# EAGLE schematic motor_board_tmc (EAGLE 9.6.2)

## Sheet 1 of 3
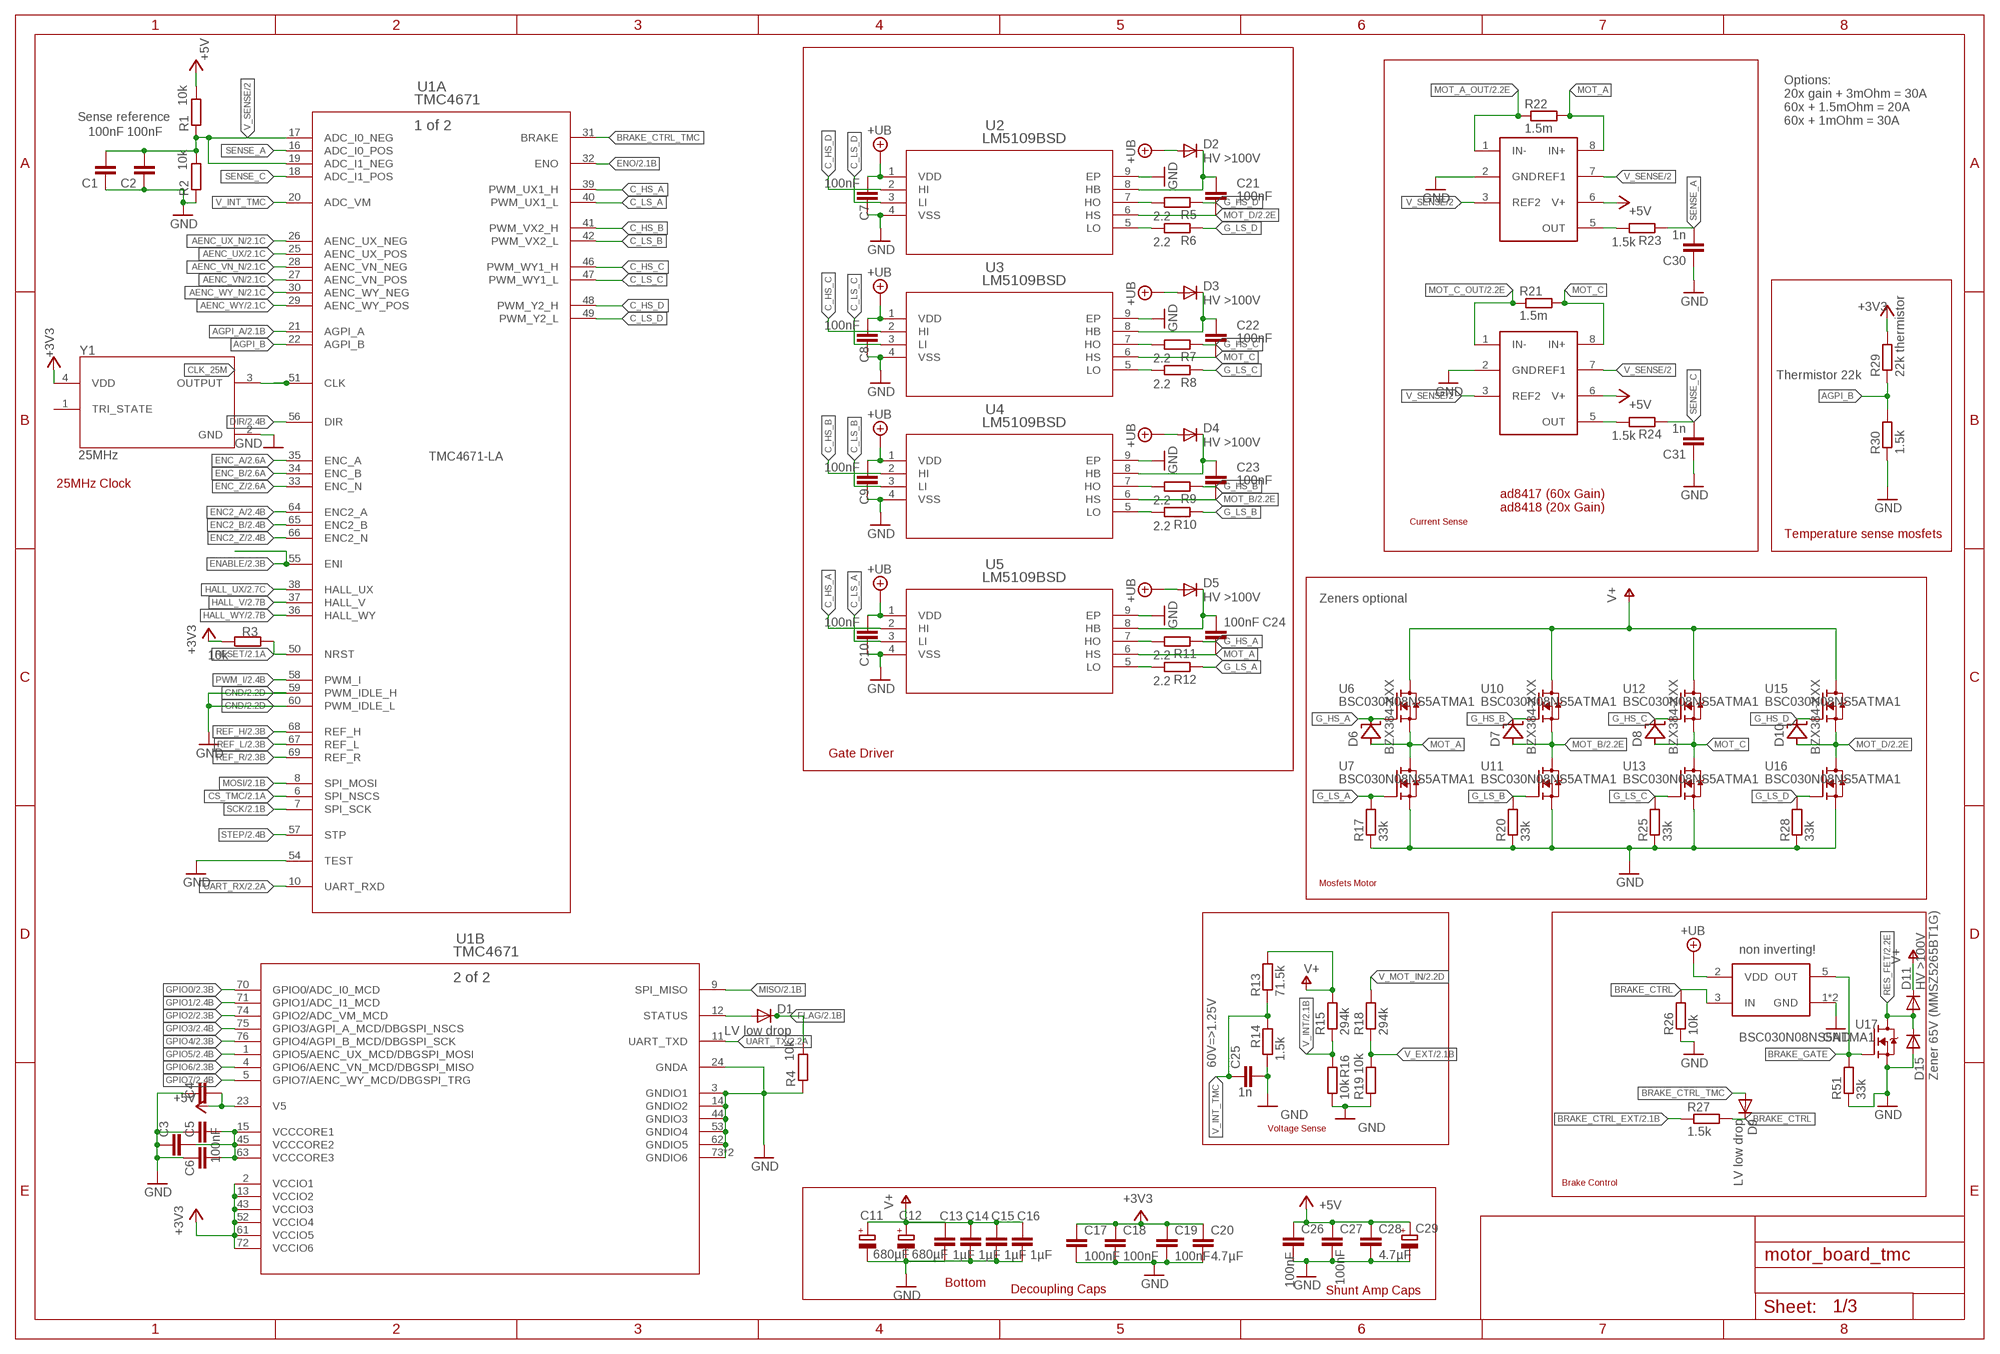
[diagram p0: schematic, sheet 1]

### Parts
C1  100nF  C-EUC0603  [C0603]
C2  100nF  C-EUC0603  [C0603]
C3  100nF  C-EUC0603  [C0603]
C4  100nF  C-EUC0603  [C0603]
C5  100nF  C-EUC0603  [C0603]
C6  100nF  C-EUC0603  [C0603]
C7  100nF  C-EUC0603  [C0603]
C8  100nF  C-EUC0603  [C0603]
C9  100nF  C-EUC0603  [C0603]
C10  100nF  C-EUC0603  [C0603]
C11  680µF  CPOL-EUE7.5-16  [E7,5-16]
C12  680µF  CPOL-EUE7.5-16  [E7,5-16]
C13  1µF  C-EUC1206  [C1206]
C14  1µF  C-EUC1206  [C1206]
C15  1µF  C-EUC1206  [C1206]
C16  1µF  C-EUC1206  [C1206]
C17  100nF  C-EUC0603  [C0603]
C18  100nF  C-EUC0603  [C0603]
C19  100nF  C-EUC0603  [C0603]
C20  4.7µF  C-EUC0805  [C0805]
C21  100nF  C-EUC0805  [C0805]
C22  100nF  C-EUC0805  [C0805]
C23  100nF  C-EUC0805  [C0805]
C24  100nF  C-EUC0805  [C0805]
C25  1n  C-EUC0603  [C0603]
C26  100nF  C-EUC0603  [C0603]
C27  100nF  C-EUC0603  [C0603]
C28  4.7µF  C-EUC0805  [C0805]
C29  CPOL-EUE5-8.5  [E5-8,5]
C30  1n  C-EUC0603  [C0603]
C31  1n  C-EUC0603  [C0603]
D1  LV low drop  DIODE_SOD-123FL  [SOD-123FL]
D2  HV >100V  DIODE_SOD-123FL  [SOD-123FL]
D3  HV >100V  DIODE_SOD-123FL  [SOD-123FL]
D4  HV >100V  DIODE_SOD-123FL  [SOD-123FL]
D5  HV >100V  DIODE_SOD-123FL  [SOD-123FL]
D6  BZX384-XXX  [SOD323-R]
D7  BZX384-XXX  [SOD323-R]
D8  BZX384-XXX  [SOD323-R]
D9  LV low drop  DIODE_SOD-123FL  [SOD-123FL]
D10  BZX384-XXX  [SOD323-R]
D11  HV >100V  DIODE_SOD-123FL  [SOD-123FL]
D15  Zener 65V (MMSZ5265BT1G)  DIODE_SOD-123FL  [SOD-123FL]
R1  10k  R-EU_R0603  [R0603]
R2  10k  R-EU_R0603  [R0603]
R3  10k  R-EU_R0603  [R0603]
R4  10k  R-EU_R0603  [R0603]
R5  2.2  R-EU_R0603  [R0603]
R6  2.2  R-EU_R0603  [R0603]
R7  2.2  R-EU_R0603  [R0603]
R8  2.2  R-EU_R0603  [R0603]
R9  2.2  R-EU_R0603  [R0603]
R10  2.2  R-EU_R0603  [R0603]
R11  2.2  R-EU_R0603  [R0603]
R12  2.2  R-EU_R0603  [R0603]
R13  71.5k  R-EU_R0805  [R0805]
R14  1.5k  R-EU_R0603  [R0603]
R15  294k  R-EU_R0805  [R0805]
R16  10k  R-EU_R0603  [R0603]
R17  33k  R-EU_R0603  [R0603]
R18  294k  R-EU_R0805  [R0805]
R19  10k  R-EU_R0603  [R0603]
R20  33k  R-EU_R0603  [R0603]
R21  1.5m  R-EU_R2512  [R2512]
R22  1.5m  R-EU_R2512  [R2512]
R23  1.5k  R-EU_R0603  [R0603]
R24  1.5k  R-EU_R0603  [R0603]
R25  33k  R-EU_R0603  [R0603]
R26  10k  R-EU_R0603  [R0603]
R27  1.5k  R-EU_R0603  [R0603]
R28  33k  R-EU_R0603  [R0603]
R29  22k thermistor  R-EU_R0603  [R0603]
R30  1.5k  R-EU_R0603  [R0603]
R51  33k  R-EU_R0603  [R0603]
U1  TMC4671  [QFN76_10P5X6P5]
U2  LM5109BSD  [SDC08A]
U3  LM5109BSD  [SDC08A]
U4  LM5109BSD  [SDC08A]
U5  LM5109BSD  [SDC08A]
U6  BSC030N08NS5ATMA1  [MOSFET_BSC093N04LSGATMA1]
U7  BSC030N08NS5ATMA1  [MOSFET_BSC093N04LSGATMA1]
U8  AD841X  [MSOP8]
U9  AD841X  [MSOP8]
U10  BSC030N08NS5ATMA1  [MOSFET_BSC093N04LSGATMA1]
U11  BSC030N08NS5ATMA1  [MOSFET_BSC093N04LSGATMA1]
U12  BSC030N08NS5ATMA1  [MOSFET_BSC093N04LSGATMA1]
U13  BSC030N08NS5ATMA1  [MOSFET_BSC093N04LSGATMA1]
U14  MCP14XX  [SOT23-5L]
U15  BSC030N08NS5ATMA1  [MOSFET_BSC093N04LSGATMA1]
U16  BSC030N08NS5ATMA1  [MOSFET_BSC093N04LSGATMA1]
U17  BSC030N08NS5ATMA1  [MOSFET_BSC093N04LSGATMA1]
Y1  25MHz  ECS-327KE-TR  [ECS-327KE-TR]

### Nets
+3V3: C17.1 C18.1 C19.1 C20.1 R3.2 R29.2 U1.2(B:VCCIO1) U1.13(B:VCCIO2) U1.43(B:VCCIO3) U1.52(B:VCCIO4) U1.61(B:VCCIO5) U1.72(B:VCCIO6) Y1.4(VDD) ; also sheet 2,3
+5V: C4.2 C26.1 C27.1 C28.1 C29.+ R1.2 U1.23(B:V5) U8.6(V+) U9.6(V+) ; also sheet 2,3
AENC_UX: U1.25(A:AENC_UX_POS) ; also sheet 2
AENC_UX_N: U1.26(A:AENC_UX_NEG) ; also sheet 2
AENC_VN: U1.27(A:AENC_VN_POS) ; also sheet 2
AENC_VN_N: U1.28(A:AENC_VN_NEG) ; also sheet 2
AENC_WY: U1.29(A:AENC_WY_POS) ; also sheet 2
AENC_WY_N: U1.30(A:AENC_WY_NEG) ; also sheet 2
AGPI_A: U1.21(A:AGPI_A) ; also sheet 2
AGPI_B: R29.1 R30.2 U1.22(A:AGPI_B)
BRAKE_CTRL: D9.C R26.2 R27.2 U14.3(IN)
BRAKE_CTRL_EXT: R27.1 ; also sheet 2
BRAKE_CTRL_TMC: D9.A U1.31(A:BRAKE)
BRAKE_GATE: R51.2 U14.5(OUT) U17.4(G)
C_HS_A: U1.39(A:PWM_UX1_H) U5.2(HI)
C_HS_B: U1.41(A:PWM_VX2_H) U4.2(HI)
C_HS_C: U1.46(A:PWM_WY1_H) U3.2(HI)
C_HS_D: U1.48(A:PWM_Y2_H) U2.2(HI)
C_LS_A: U1.40(A:PWM_UX1_L) U5.3(LI)
C_LS_B: U1.42(A:PWM_VX2_L) U4.3(LI)
C_LS_C: U1.47(A:PWM_WY1_L) U3.3(LI)
C_LS_D: U1.49(A:PWM_Y2_L) U2.3(LI)
CLK_25M: U1.51(A:CLK) Y1.3(OUTPUT)
CS_TMC: U1.6(A:SPI_NSCS) ; also sheet 2
DIR: U1.56(A:DIR) ; also sheet 2
ENABLE: U1.55(A:ENI) ; also sheet 2
ENC2_A: U1.64(A:ENC2_A) ; also sheet 2
ENC2_B: U1.65(A:ENC2_B) ; also sheet 2
ENC2_Z: U1.66(A:ENC2_N) ; also sheet 2
ENC_A: U1.35(A:ENC_A) ; also sheet 2
ENC_B: U1.34(A:ENC_B) ; also sheet 2
ENC_Z: U1.33(A:ENC_N) ; also sheet 2
ENO: U1.32(A:ENO) ; also sheet 2
FLAG: D1.C R4.2 ; also sheet 2
G_HS_A: D6.C R11.1 U6.4(G)
G_HS_B: D7.C R9.1 U10.4(G)
G_HS_C: D8.C R7.1 U12.4(G)
G_HS_D: D10.C R5.1 U15.4(G)
G_LS_A: R12.1 R17.2 U7.4(G)
G_LS_B: R10.1 R20.2 U11.4(G)
G_LS_C: R8.1 R25.2 U13.4(G)
G_LS_D: R6.1 R28.2 U16.4(G)
GND: C1.1 C2.1 C3.1 C4.1 C5.1 C6.1 C7.1 C8.1 C9.1 C10.1 C11.- C12.- C13.2 C14.2 C15.2 C16.2 C17.2 C18.2 C19.2 C20.2 C25.2 C26.2 C27.2 C28.2 C29.- C30.1 C31.1 D15.A R2.1 R4.1 R14.1 R16.1 R17.1 R19.1 R20.1 R25.1 R26.1 R28.1 R30.1 R51.1 U1.3(B:GNDIO1) U1.14(B:GNDIO2) U1.24(B:GNDA) U1.44(B:GNDIO3) U1.53(B:GNDIO4) U1.54(A:TEST) U1.59(A:PWM_IDLE_H) U1.60(A:PWM_IDLE_L) U1.62(B:GNDIO5) U1.73(B:GNDIO6) U1.77(B:GNDIO6) U2.4(VSS) U2.9(EP) U3.4(VSS) U3.9(EP) U4.4(VSS) U4.9(EP) U5.4(VSS) U5.9(EP) U7.1(S) U7.2(S) U7.3(S) U8.2(GND) U9.2(GND) U11.1(S) U11.2(S) U11.3(S) U13.1(S) U13.2(S) U13.3(S) U14.1(GND) U14.4(GND) U16.1(S) U16.2(S) U16.3(S) U17.1(S) U17.2(S) U17.3(S) Y1.2(GND) ; also sheet 2,3
GPIO0: U1.70(B:GPIO0/ADC_I0_MCD) ; also sheet 2
GPIO1: U1.71(B:GPIO1/ADC_I1_MCD) ; also sheet 2
GPIO2: U1.74(B:GPIO2/ADC_VM_MCD) ; also sheet 2
GPIO3: U1.75(B:GPIO3/AGPI_A_MCD/DBGSPI_NSCS) ; also sheet 2
GPIO4: U1.76(B:GPIO4/AGPI_B_MCD/DBGSPI_SCK) ; also sheet 2
GPIO5: U1.1(B:GPIO5/AENC_UX_MCD/DBGSPI_MOSI) ; also sheet 2
GPIO6: U1.4(B:GPIO6/AENC_VN_MCD/DBGSPI_MISO) ; also sheet 2
GPIO7: U1.5(B:GPIO7/AENC_WY_MCD/DBGSPI_TRG) ; also sheet 2
HALL_UX: U1.38(A:HALL_UX) ; also sheet 2
HALL_V: U1.37(A:HALL_V) ; also sheet 2
HALL_WY: U1.36(A:HALL_WY) ; also sheet 2
MISO: U1.9(B:SPI_MISO) ; also sheet 2
MOSI: U1.8(A:SPI_MOSI) ; also sheet 2
MOT_A: C24.2 D6.A R22.2 U5.6(HS) U6.1(S) U6.2(S) U6.3(S) U7.5(D) U8.8(IN+)
MOT_A_OUT: R22.1 U8.1(IN-) ; also sheet 2
MOT_B: C23.2 D7.A U4.6(HS) U10.1(S) U10.2(S) U10.3(S) U11.5(D) ; also sheet 2
MOT_C: C22.2 D8.A R21.2 U3.6(HS) U9.8(IN+) U12.1(S) U12.2(S) U12.3(S) U13.5(D)
MOT_C_OUT: R21.1 U9.1(IN-) ; also sheet 2
MOT_D: C21.2 D10.A U2.6(HS) U15.1(S) U15.2(S) U15.3(S) U16.5(D) ; also sheet 2
N$4: D1.A U1.12(B:STATUS)
N$6: R23.2 U8.5(OUT)
N$10: R24.2 U9.5(OUT)
N$13: R12.2 U5.5(LO)
N$18: C24.1 D5.C U5.8(HB)
N$27: R11.2 U5.7(HO)
N$28: C23.1 D4.C U4.8(HB)
N$29: R10.2 U4.5(LO)
N$30: R9.2 U4.7(HO)
N$31: C21.1 D2.C U2.8(HB)
N$32: R6.2 U2.5(LO)
N$33: R5.2 U2.7(HO)
N$34: C22.1 D3.C U3.8(HB)
N$35: R8.2 U3.5(LO)
N$36: R7.2 U3.7(HO)
PWM_I: U1.58(A:PWM_I) ; also sheet 2
REF_H: U1.68(A:REF_H) ; also sheet 2
REF_L: U1.67(A:REF_L) ; also sheet 2
REF_R: U1.69(A:REF_R) ; also sheet 2
RES_FET: D11.A D15.C U17.5(D) ; also sheet 2
RESET: R3.1 U1.50(A:NRST) ; also sheet 2
SCK: U1.7(A:SPI_SCK) ; also sheet 2
SENSE_A: C30.2 R23.1 U1.16(A:ADC_I0_POS)
SENSE_C: C31.2 R24.1 U1.18(A:ADC_I1_POS)
STEP: U1.57(A:STP) ; also sheet 2
UART_RX: U1.10(A:UART_RXD) ; also sheet 2
UART_TX: U1.11(B:UART_TXD) ; also sheet 2
V+: C11.+ C12.+ C13.1 C14.1 C15.1 C16.1 D11.C R13.2 R15.2 U6.5(D) U10.5(D) U12.5(D) U15.5(D) ; also sheet 2,3
V_EXT: R18.1 R19.2 ; also sheet 2
V_GD: C7.2 C8.2 C9.2 C10.2 D2.A D3.A D4.A D5.A U2.1(VDD) U3.1(VDD) U4.1(VDD) U5.1(VDD) U14.2(VDD) ; supply symbol labelled +UB ; also sheet 2,3
V_INT: R15.1 R16.2 ; also sheet 2
V_INT_TMC: C25.1 R13.1 R14.2 U1.20(A:ADC_VM)
V_MOT_IN: R18.2 ; also sheet 2,3
V_SENSE/2: C1.2 C2.2 R1.1 R2.2 U1.17(A:ADC_I0_NEG) U1.19(A:ADC_I1_NEG) U8.3(REF2) U8.7(REF1) U9.3(REF2) U9.7(REF1)
VCORE: C3.2 C5.2 C6.2 U1.15(B:VCCCORE1) U1.45(B:VCCCORE2) U1.63(B:VCCCORE3)
Unconnected: Y1.1(TRI_STATE)

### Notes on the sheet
- Sense reference
- Options:
  20x gain + 3mOhm = 30A
  60x + 1.5mOhm = 20A
  60x + 1mOhm = 30A
- Thermistor 22k
- TMC4671-LA
- 25MHz Clock
- Current Sense
- ad8417 (60x Gain)
  ad8418 (20x Gain)
- Temperature sense mosfets
- Zeners optional
- Gate Driver
- Mosfets Motor
- non inverting!
- 60V=>1.25V
- Voltage Sense
- Brake Control
- Bottom
- Decoupling Caps | Shunt Amp Caps

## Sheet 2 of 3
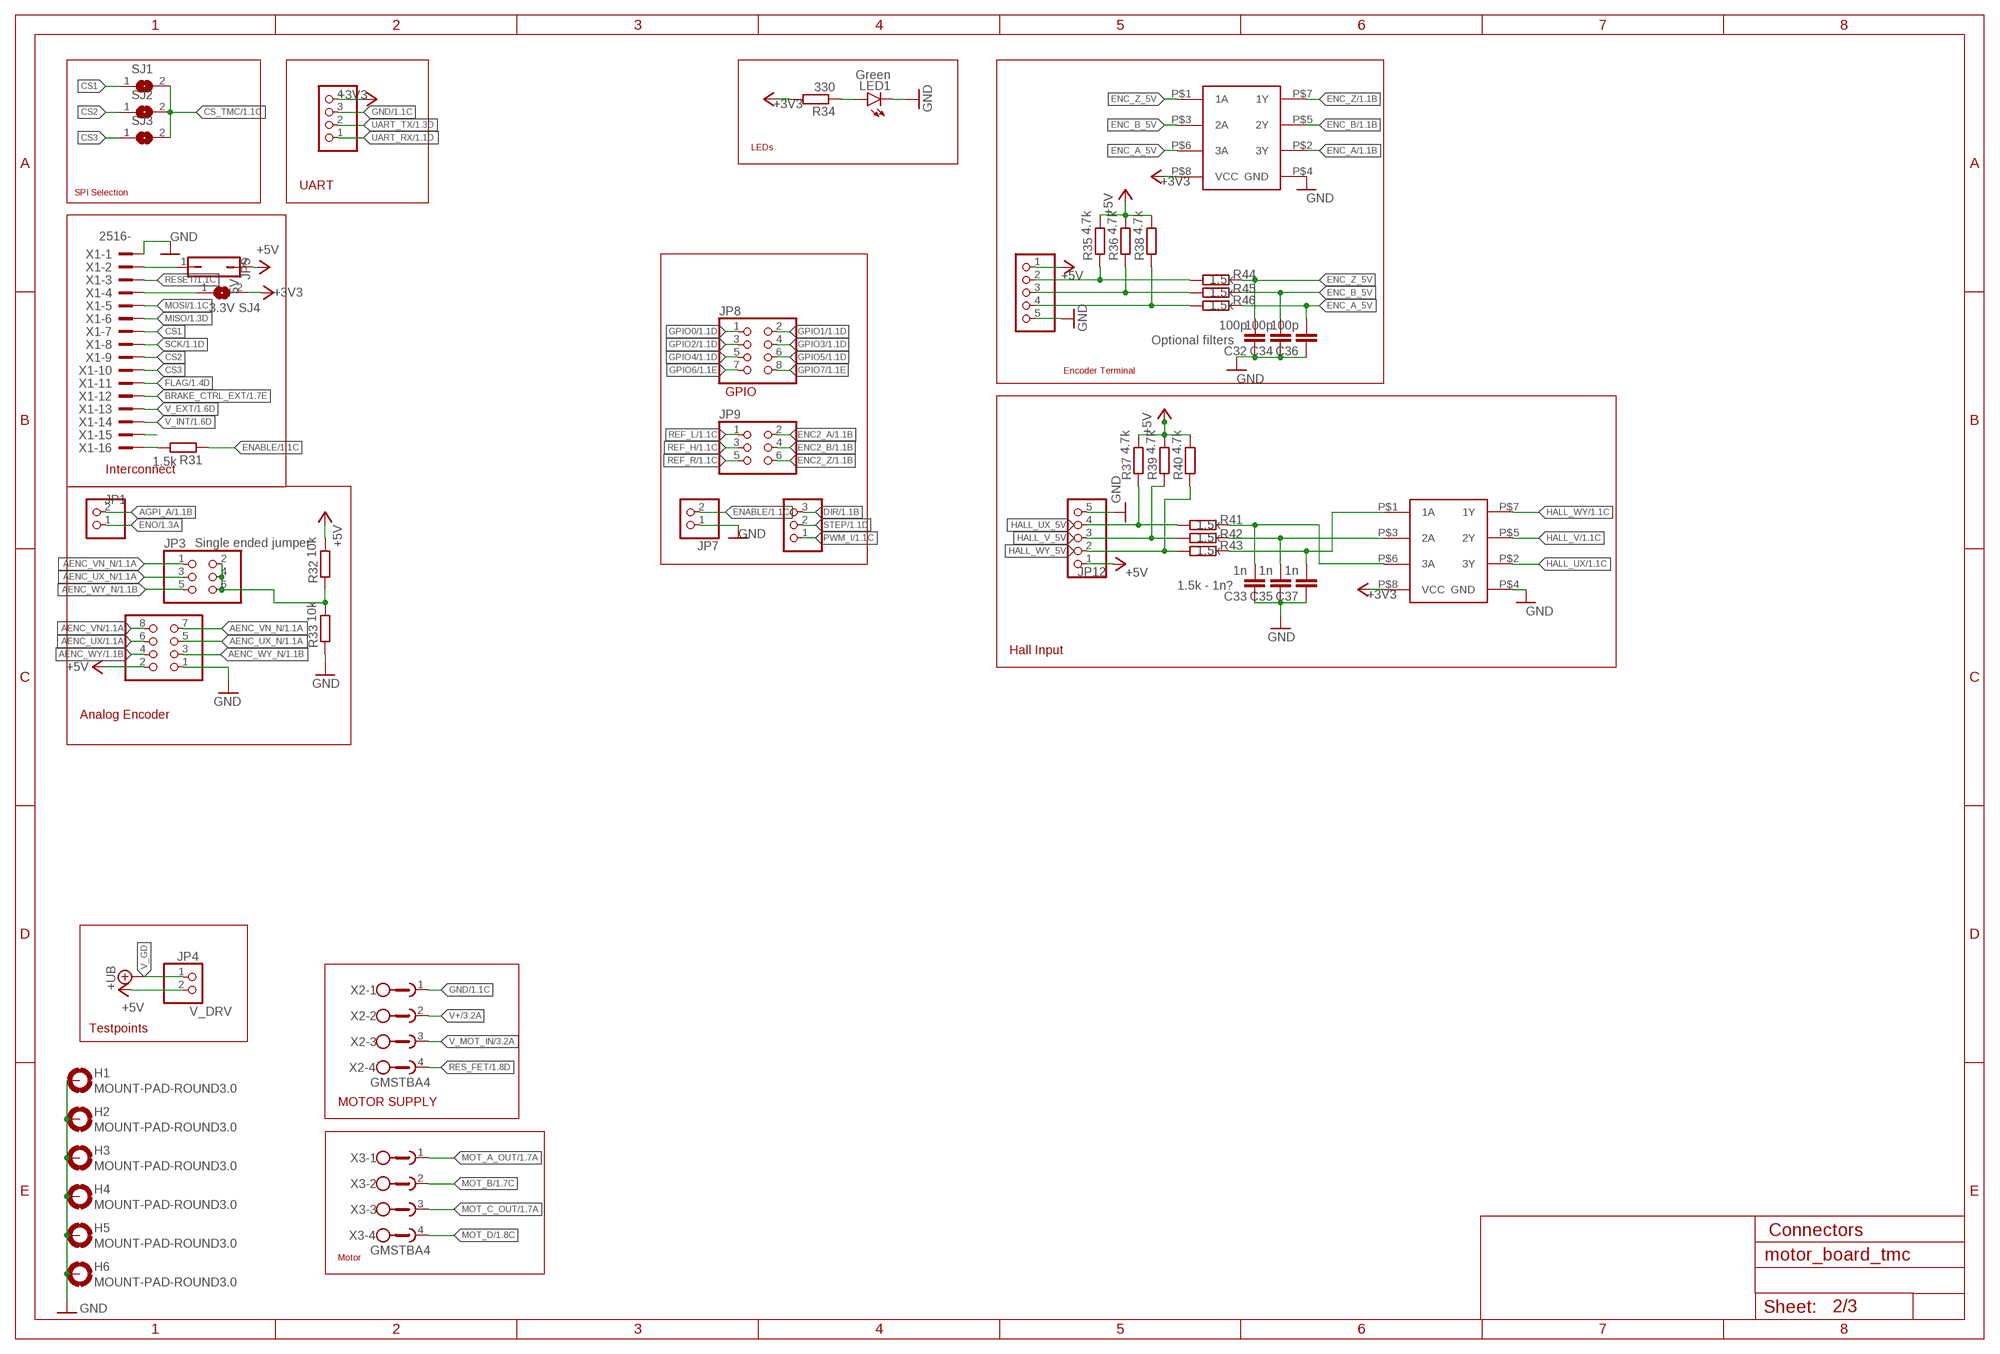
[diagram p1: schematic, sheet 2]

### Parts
C32  100p  C-EUC0603  [C0603]
C33  1n  C-EUC0603  [C0603]
C34  100p  C-EUC0603  [C0603]
C35  1n  C-EUC0603  [C0603]
C36  100p  C-EUC0603  [C0603]
C37  1n  C-EUC0603  [C0603]
H1  MOUNT-PAD-ROUND3.0  [3,0-PAD]
H2  MOUNT-PAD-ROUND3.0  [3,0-PAD]
H3  MOUNT-PAD-ROUND3.0  [3,0-PAD]
H4  MOUNT-PAD-ROUND3.0  [3,0-PAD]
H5  MOUNT-PAD-ROUND3.0  [3,0-PAD]
H6  MOUNT-PAD-ROUND3.0  [3,0-PAD]
JP1  PINHD-1X2  [1X02]
JP2  PINHD-2X4  [2X04]
JP3  PINHD-2X3  [2X03]
JP4  V_DRV  PINHD-1X2  [1X02]
JP5  5V  JP1Q  [JP1]
JP6  PINHD-1X4  [1X04]
JP7  PINHD-1X2  [1X02]
JP8  PINHD-2X4  [2X04]
JP9  PINHD-2X3  [2X03]
JP10  PINHD-1X3  [1X03]
JP11  PINHD-1X5  [1X05]
JP12  PINHD-1X5  [1X05]
LED1  Green  LEDSML0805  [SML0805]
R31  1.5k  R-EU_R0603  [R0603]
R32  10k  R-EU_R0603  [R0603]
R33  10k  R-EU_R0603  [R0603]
R34  330  R-EU_R0603  [R0603]
R35  4.7k  R-EU_R0603  [R0603]
R36  4.7k  R-EU_R0603  [R0603]
R37  4.7k  R-EU_R0603  [R0603]
R38  4.7k  R-EU_R0603  [R0603]
R39  4.7k  R-EU_R0603  [R0603]
R40  4.7k  R-EU_R0603  [R0603]
R41  1.5k  R-EU_R0603  [R0603]
R42  1.5k  R-EU_R0603  [R0603]
R43  1.5k  R-EU_R0603  [R0603]
R44  1.5k  R-EU_R0603  [R0603]
R45  1.5k  R-EU_R0603  [R0603]
R46  1.5k  R-EU_R0603  [R0603]
SJ1  SJ  [SJ]
SJ2  SJ  [SJ]
SJ3  SJ  [SJ]
SJ4  3.3V  SJ  [SJ]
U18  NC7NZ17K8X-3-BUFFER  [VFSOP-8]
U19  NC7NZ17K8X-3-BUFFER  [VFSOP-8]
X1  2516-  [PAK100/2500-16]
X2  GMSTBA4  [GMSTBA4]
X3  GMSTBA4  [GMSTBA4]

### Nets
+3V3: JP6.4 R34.2 SJ4.2 U18.P$8(VCC) U19.P$8(VCC) ; also sheet 1,3
+5V: JP2.2 JP4.2 JP5.2 JP11.1 JP12.1 R32.2 R35.2 R36.2 R37.2 R38.2 R39.2 R40.2 ; also sheet 1,3
AENC_UX: JP2.6 ; also sheet 1
AENC_UX_N: JP2.5 JP3.3 ; also sheet 1
AENC_VN: JP2.8 ; also sheet 1
AENC_VN_N: JP2.7 JP3.1 ; also sheet 1
AENC_WY: JP2.4 ; also sheet 1
AENC_WY_N: JP2.3 JP3.5 ; also sheet 1
AGPI_A: JP1.2 ; also sheet 1
BRAKE_CTRL_EXT: X1.12 ; also sheet 1
CS1: SJ1.1 X1.7
CS2: SJ2.1 X1.9
CS3: SJ3.1 X1.10
CS_TMC: SJ1.2 SJ2.2 SJ3.2 ; also sheet 1
DIR: JP10.3 ; also sheet 1
ENABLE: JP7.2 R31.1 ; also sheet 1
ENC2_A: JP9.2 ; also sheet 1
ENC2_B: JP9.4 ; also sheet 1
ENC2_Z: JP9.6 ; also sheet 1
ENC_A: U18.P$2(3Y) ; also sheet 1
ENC_A_5V: C36.2 R46.1 U18.P$6(3A)
ENC_B: U18.P$5(2Y) ; also sheet 1
ENC_B_5V: C34.2 R45.1 U18.P$3(2A)
ENC_Z: U18.P$7(1Y) ; also sheet 1
ENC_Z_5V: C32.2 R44.1 U18.P$1(1A)
ENO: JP1.1 ; also sheet 1
FLAG: X1.11 ; also sheet 1
GND: C32.1 C33.1 C34.1 C35.1 C36.1 C37.1 H1.B3,0(MOUNT) H2.B3,0(MOUNT) H3.B3,0(MOUNT) H4.B3,0(MOUNT) H5.B3,0(MOUNT) H6.B3,0(MOUNT) JP2.1 JP6.3 JP7.1 JP11.5 JP12.5 LED1.C R33.1 U18.P$4(GND) U19.P$4(GND) X1.1 X2.1 ; also sheet 1,3
GPIO0: JP8.1 ; also sheet 1
GPIO1: JP8.2 ; also sheet 1
GPIO2: JP8.3 ; also sheet 1
GPIO3: JP8.4 ; also sheet 1
GPIO4: JP8.5 ; also sheet 1
GPIO5: JP8.6 ; also sheet 1
GPIO6: JP8.7 ; also sheet 1
GPIO7: JP8.8 ; also sheet 1
HALL_UX: U19.P$2(3Y) ; also sheet 1
HALL_UX_5V: C33.2 R41.1 U19.P$6(3A)
HALL_V: U19.P$5(2Y) ; also sheet 1
HALL_V_5V: C35.2 R42.1 U19.P$3(2A)
HALL_WY: U19.P$7(1Y) ; also sheet 1
HALL_WY_5V: C37.2 R43.1 U19.P$1(1A)
MISO: X1.6 ; also sheet 1
MOSI: X1.5 ; also sheet 1
MOT_A_OUT: X3.1 ; also sheet 1
MOT_B: X3.2 ; also sheet 1
MOT_C_OUT: X3.3 ; also sheet 1
MOT_D: X3.4 ; also sheet 1
N$1: JP12.4 R37.1 R41.2
N$2: X1.15
N$3: JP12.3 R39.1 R42.2
N$7: JP11.4 R38.1 R46.2
N$8: LED1.A R34.1
N$9: JP11.3 R36.1 R45.2
N$11: JP11.2 R35.1 R44.2
N$15: JP12.2 R40.1 R43.2
N$17: R31.2 X1.16
N$20: SJ4.1 X1.4
N$22: JP3.2 JP3.4 JP3.6 R32.1 R33.2
N$23: JP5.1 X1.2
PWM_I: JP10.1 ; also sheet 1
REF_H: JP9.3 ; also sheet 1
REF_L: JP9.1 ; also sheet 1
REF_R: JP9.5 ; also sheet 1
RES_FET: X2.4 ; also sheet 1
RESET: X1.3 ; also sheet 1
SCK: X1.8 ; also sheet 1
STEP: JP10.2 ; also sheet 1
UART_RX: JP6.1 ; also sheet 1
UART_TX: JP6.2 ; also sheet 1
V+: X2.2 ; also sheet 1,3
V_EXT: X1.13 ; also sheet 1
V_GD: JP4.1 ; supply symbol labelled +UB ; also sheet 1,3
V_INT: X1.14 ; also sheet 1
V_MOT_IN: X2.3 ; also sheet 1,3

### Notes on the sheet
- LEDs
- UART
- SPI Selection
- Optional filters
- Encoder Terminal
- GPIO
- Interconnect
- Single ended jumper
- 1.5k - 1n?
- Hall Input
- Analog Encoder
- Testpoints
- MOTOR SUPPLY
- Connectors
- Motor

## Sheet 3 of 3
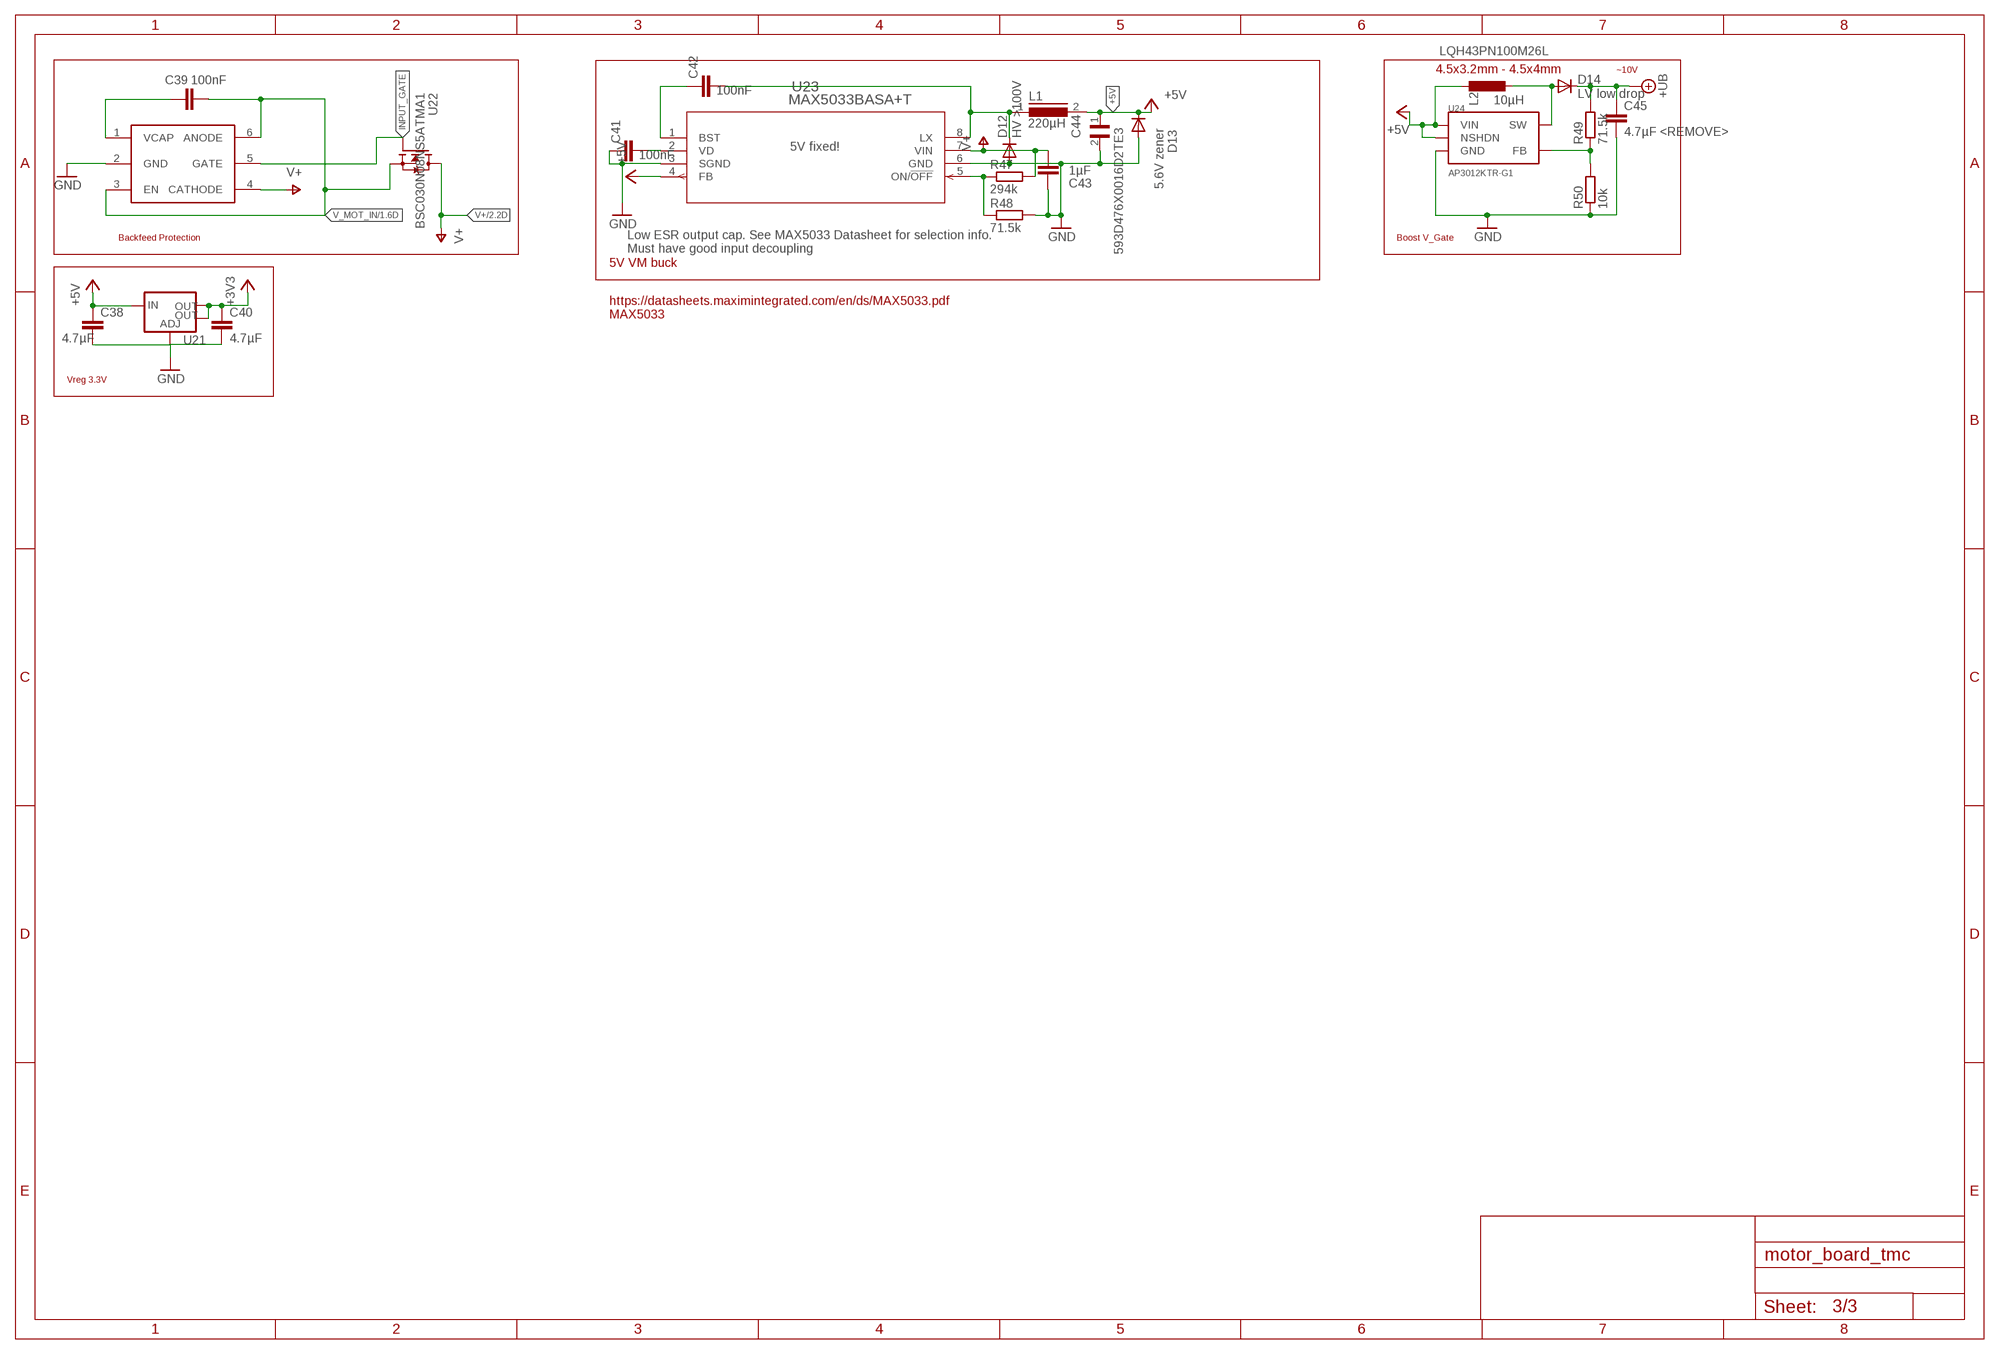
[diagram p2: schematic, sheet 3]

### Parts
C38  4.7µF  C-EUC0805  [C0805]
C39  100nF  C-EUC0805  [C0805]
C40  4.7µF  C-EUC0805  [C0805]
C41  100nF  C-EUC0603  [C0603]
C42  100nF  C-EUC0603  [C0603]
C43  1µF  C-EUC1206  [C1206]
C44  593D476X0016D2TE3  [CAPPM7343X310N]
C45  4.7µF <REMOVE>  C-EUC0805  [C0805]
D12  HV >100V  DIODE_SOD-123FL  [SOD-123FL]
D13  5.6V zener  DIODE_SOD-123FL  [SOD-123FL]
D14  LV low drop  DIODE_SOD-123FL  [SOD-123FL]
L1  220µH  8MMINDUCTOR  [8MMINDUCTOR]
L2  10µH  L-EUL4532P  [L4532P]
R47  294k  R-EU_R0805  [R0805]
R48  71.5k  R-EU_R0805  [R0805]
R49  71.5k  R-EU_R0805  [R0805]
R50  10k  R-EU_R0603  [R0603]
U20  LM74700-Q1  [SOT23-6]
U21  V_REG_LM1117SOT223  [SOT223]
U22  BSC030N08NS5ATMA1  [MOSFET_BSC093N04LSGATMA1]
U23  MAX5033BASA+T  [21-0041B_8_MXM]
U24  AP3012KTR-G1  [SOT23-5L]

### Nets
+3V3: C40.1 U21.2(OUT) U21.4(OUT) ; also sheet 1,2
+5V: C38.1 C44.1 D13.C L1.2 L2.1 U21.3(IN) U23.4(FB) U24.4(NSHDN) U24.5(VIN) ; also sheet 1,2
GND: C38.2 C40.2 C41.1 C43.1 C44.2 C45.2 D12.A D13.A R48.2 R50.1 U20.2(GND) U21.1(ADJ) U23.3(SGND) U23.6(GND) U24.2(GND) ; also sheet 1,2
INPUT_GATE: U20.5(GATE) U22.4(G)
N$5: R49.1 R50.2 U24.3(FB)
N$12: D14.A L2.2 U24.1(SW)
N$16: C42.2 D12.C L1.1 U23.8(LX)
N$19: C42.1 U23.1(BST)
N$21: R47.1 R48.1 U23.5(ON/!OFF)
N$24: C39.1 U20.1(VCAP)
N$25: C41.2 U23.2(VD)
V+: C43.2 R47.2 U20.4(CATHODE) U22.5(D) U23.7(VIN) ; also sheet 1,2
V_GD: C45.1 D14.C R49.2 ; supply symbol labelled +UB ; also sheet 1,2
V_MOT_IN: C39.2 U20.3(EN) U20.6(ANODE) U22.1(S) U22.2(S) U22.3(S) ; also sheet 1,2

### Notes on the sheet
- LQH43PN100M26L
- 4.5x3.2mm - 4.5x4mm | ~10V
- 5V fixed!
- Backfeed Protection | Boost V_Gate
- Low ESR output cap. See MAX5033 Datasheet for selection info.
  Must have good input decoupling
- 5V VM buck
- https://datasheets.maximintegrated.com/en/ds/MAX5033.pdf
  MAX5033
- Vreg 3.3V

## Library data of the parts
C1-C10 C13-C28 C30-C43 C45 = resistor:C-EU: CAPACITOR, European symbol
C11 C12 C29 = resistor:CPOL-EU: POLARIZED CAPACITOR, European symbol
C44 = Powermisc:593D476X0016D2TE3: 593D Series 47 uF ±20% 16 V Surface Mount Molded Solid Tantalum Capacitor; ARROW_ELECTRONICS-PURCHASE-URL: https://snapeda.com/shop?store=Arrow+Electronics&id=1736527; DESCRIPTION: 47µF Molded Tantalum Capacitors 16V 2917 (7343 Metric) 150mOhm; DIGI-KEY_PART_NUMBER: 718-2142-1-ND; MF: Vishay Sprague; MOUSER-PURCHASE-URL: https://snapeda.com/shop?store=Mouser&id=1736527; MP: 593D476X0016D2TE3; PACKAGE: 2917 Vishay
D1-D5 D9 D11-D15 = adafruit:DIODE: Diode
D6-D8 D10 = Powermisc:BZX384-XXX
H1-H6 = holes:MOUNT-PAD-ROUND: MOUNTING PAD, round
JP1 JP4 JP7 = pinhead:PINHD-1X2: PIN HEADER
JP2 JP8 = pinhead:PINHD-2X4: PIN HEADER
JP3 JP9 = pinhead:PINHD-2X3: PIN HEADER
JP5 = jumper:JP1Q: JUMPER
JP6 = pinhead:PINHD-1X4: PIN HEADER
JP10 = pinhead:PINHD-1X3: PIN HEADER
JP11 JP12 = pinhead:PINHD-1X5: PIN HEADER
L1 = Powermisc:8MMINDUCTOR: Inductor; SPICEPREFIX: L
L2 = rcl:L-EU: INDUCTOR, European symbol; SPICEPREFIX: L
LED1 = led:LED: LED
R1-R51 = resistor:R-EU_: RESISTOR, European symbol
SJ1-SJ4 = jumper:SJ: SMD solder JUMPER
U1 = Trinamic:TMC4671; MANUFACTURER_PART_NUMBER: TMC4671ES; VENDOR: TRINAMIC
U2-U5 = Powermisc:LM5109BSD; MANUFACTURER_PART_NUMBER: lm5109bsd; VENDOR: Texas Instruments
U6 U7 U10-U13 U15-U17 U22 = OHSC_Power:BSC030N08NS5ATMA1: None; AVAILABILITY: Unavailable; DESCRIPTION: N-Channel 80 V 100 A 3 mO 61 nC SMT OptiMOS Power Mosfet - SuperSO-8; MF: Infineon Technologies; MP: BSC030N08NS5ATMA1; PACKAGE: PowerTDFN-8 Infineon; PRICE: None
U8 U9 = Powermisc:AD841X
U14 = Powermisc:MCP14XX
U18 U19 = Powermisc:NC7NZ17K8X-3-BUFFER
U20 = OHSC_Power:LM74700-Q1
U21 = SparkFun-IC-Power:V_REG_LM1117: Voltage Regulator LM1117 Standard adjustable voltage regulator but in SMD form. Spark Fun Electronics SKU : COM-00595; PROD_ID: VREG-08170
U23 = Powermisc:MAX5033BASA+T; BUILT_BY: EMA_UL_Team; MANUFACTURER_PART_NUMBER: max5033basa+T; SOURCELIBRARY: Maxim_2014-06-20; VENDOR: Maxim Integrated Products
U24 = Powermisc:AP3012KTR-G1
X1 = con-3m:2516-: 3M (TM) Pak 100 4-Wall Header Source: 3M; OC_FARNELL: unknown; OC_NEWARK: unknown
X2 X3 = con-phoenix-762:GMSTBA4: PHOENIX; MF: FARNELL; MPN: 1757268; OC_FARNELL: 3705195; OC_NEWARK: 71C4163
Y1 = Crystals:ECS-327KE-TR: XTAL OSC XO 32.7680KHZ CMOS SMD Manufacturer's datasheet; CREATED_BY: PCBLayout.com; DIGIKEY_PART_NUMBER: XC1751TR-ND; MANUFACTURER: ECS Inc.; MPN: ECS-327KE-TR; PACKAGE: 4-SMD

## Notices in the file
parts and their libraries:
SparkFun-IC-Power: Licensing: Creative Commons ShareAlike 4.0 International - https://creativecommons.org/licenses/by-sa/4.0
